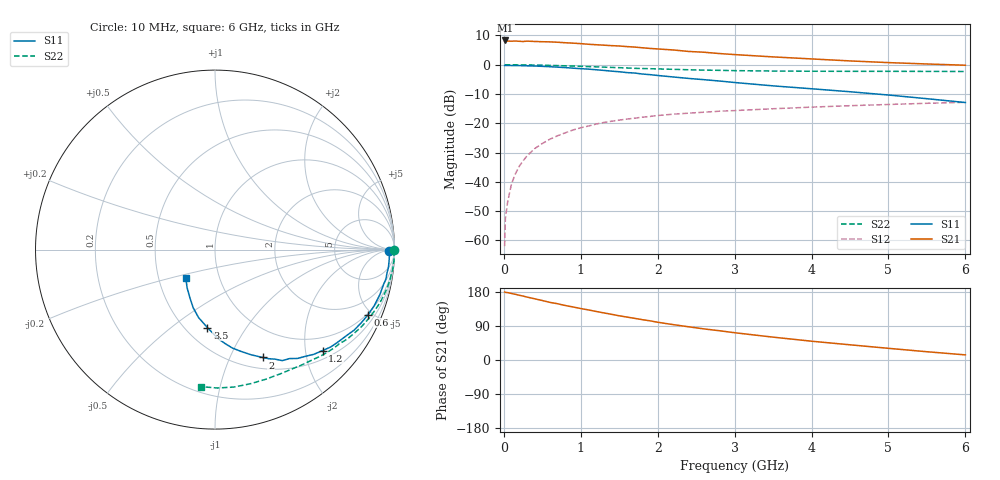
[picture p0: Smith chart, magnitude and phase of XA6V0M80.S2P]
! SIEMENS Discrete & RF Semiconductors
! BFY180
! Si NPN RF Bipolar Junction Transistor in MICRO-X
! VCE = 6 V  IC = 0.8 mA
! Common Emitter S-Parameters:  May  1997
# GHz  S  MA  R  50
!  f  S11  S21  S12  S22
! GHz  MAG  ANG  MAG  ANG  MAG  ANG  MAG  ANG
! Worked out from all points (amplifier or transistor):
!   36 points, 10 MHz to 6 GHz, reference 50 ohm
!   highest |S21| = 8.3 dB at 20 MHz (marker M1)
!   |S21| within 3 dB of that: start of sweep to 2.059 GHz
!   unconditionally stable (mu >= 1): 4.677 GHz to end of sweep
!   at 250 MHz: K = 0.04, MSG = 20.4 dB, |S12| = -32.8 dB
!   at 1.4 GHz: K = 0.44, MSG = 12.9 dB, |S12| = -19.3 dB
!   at 6 GHz: K = 1.04, MAG = 5.2 dB, |S12| = -12.8 dB
!   S11 on the Smith chart (normalised r, x): 10 MHz: 67, -12; 600 MHz: 0.92, -4.74; 1.2 GHz: 0.68, -2.36; 2 GHz: 0.63, -1.33; 3.5 GHz: 0.63, -0.68; 6 GHz: 0.69, -0.23
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0.01  0.9716 -0.3  2.531 179.4  0.0008 91.7  0.9987 -0.2
0.02  0.9756 -0.9  2.602 178.6  0.0024 88.7  0.9991 -0.5
0.05  0.9722 -1.8  2.538 177.8  0.0046 85.5  0.9989 -1.2
0.1  0.972 -3.9  2.527 175.5  0.0093 91.1  0.998 -2.6
0.2  0.9674 -7.6  2.518 170.8  0.0185 84.3  0.9959 -5.0
0.3  0.9594 -11.6  2.534 166.1  0.0277 81.9  0.9929 -7.4
0.4  0.9522 -15.3  2.501 161.6  0.037 78.7  0.9895 -9.8
0.6  0.927 -23.0  2.462 152.0  0.0537 73.6  0.9754 -14.6
0.8  0.8949 -30.2  2.378 143.7  0.0691 68.1  0.9597 -19.2
1.1  0.8432 -40.0  2.241 132.1  0.09 60.6  0.9314 -25.6
1.2  0.8222 -43.2  2.2 128.1  0.0973 58.3  0.9226 -27.7
1.5  0.7605 -52.9  2.095 116.7  0.1136 52.1  0.8922 -33.5
1.7  0.7232 -58.8  2.008 110.0  0.1223 48.6  0.8696 -36.9
2  0.6567 -66.2  1.864 99.6  0.1361 43.9  0.8505 -41.8
2.2  0.6194 -71.1  1.791 93.4  0.1433 40.8  0.8365 -45.0
2.6  0.5569 -80.0  1.638 82.1  0.1549 35.8  0.8114 -50.7
3  0.4981 -87.8  1.493 72.0  0.1652 31.4  0.7944 -56.1
3.5  0.4364 -95.6  1.363 60.3  0.1776 26.8  0.782 -62.3
4  0.3896 -103.6  1.259 49.6  0.1892 22.4  0.7755 -68.8
4.5  0.3464 -110.5  1.164 40.1  0.2003 18.3  0.773 -75.3
5.5  0.2636 -126.1  1.032 21.8  0.2201 10.2  0.7712 -89.0
6  0.2267 -136.0  0.982 13.5  0.2286 5.7  0.7675 -95.9
